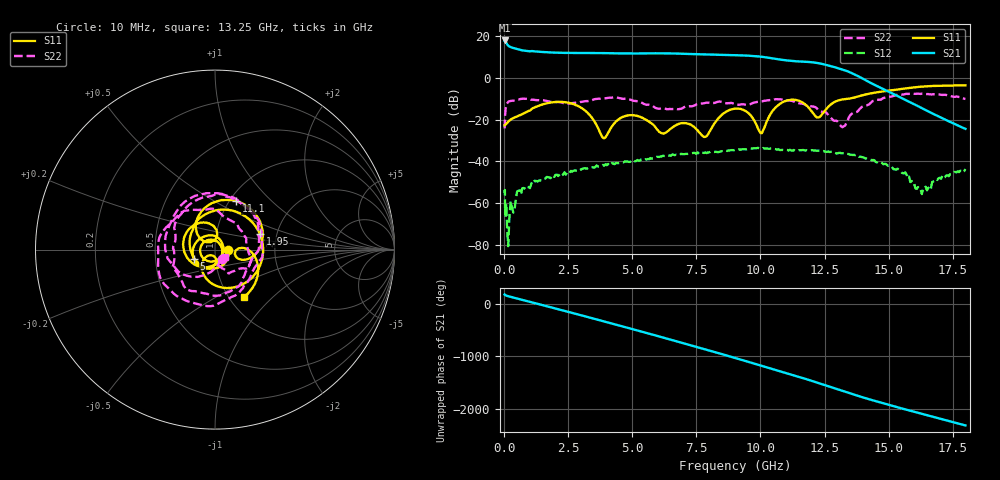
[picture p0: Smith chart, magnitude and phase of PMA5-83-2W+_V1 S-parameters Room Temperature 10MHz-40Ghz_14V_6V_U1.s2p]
!Mini-Circuits Laboratory
!S-Parameters
!Model: US-AMP-1
!Run / Lot / Date Code: N/A /  / N/A
!Fixture: ON TB-
!Network Analyzer: NFA N8975A;  Serial number: 74408
!Date: 12/1/2023 at 8:03:47 AM
!No.: Unit# 1 (#1)
!Tested with:
!Condition 4: Vdd = +14V; Vg2= +6V; Idd= 400mA
# Hz  S  dB  R  50
!Frequency  S11 dB  S11 Deg  S21 dB  S21 Deg  S12 dB  S12 Deg  S22 dB  S22 Deg
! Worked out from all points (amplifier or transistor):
!   368 points, 10 MHz to 18 GHz, reference 50 ohm
!   highest |S21| = 18.0 dB at 20 MHz (marker M1)
!   |S21| within 3 dB of that: start of sweep to 215.1 MHz
!   unconditionally stable (mu >= 1): start of sweep to end of sweep
!   at 2.7 GHz: K = 18.48, MAG = 12.5 dB, |S12| = -44.4 dB
!   at 8.85 GHz: K = 6.93, MAG = 11.4 dB, |S12| = -34.6 dB
!   at 18 GHz: K = 621.43, MAG = -21.3 dB, |S12| = -43.6 dB
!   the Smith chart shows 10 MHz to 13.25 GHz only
!   S11 on the Smith chart (normalised r, x): 10 MHz: 1.16, -0.00; 1.95 GHz: 1.64, +0.30; 5 GHz: 0.78, -0.08; 11.1 GHz: 1.07, +0.64; 13.25 GHz: 1.18, -0.68
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1e7  -22.71 -0.8  17.78 177.5  -55.13 12.2  -24.12 -54.2
2e7  -22.66 -4.0  17.98 174.2  -53.64 12.2  -20.38 -83.6
5e8  -18.43 -141.9  13.87 101.3  -54.33 60.9  -10.56 141.3
1.1e9  -14.54 124.1  12.89 26.5  -49.30 -38.3  -10.36 74.3
1.95e9  -11.53 18.7  12.15 -82.2  -47.38 -143.6  -11.66 1.0
2.55e9  -11.99 -46.9  12.01 -158.9  -45.44 143.8  -12.18 -34.4
3.05e9  -14.67 -98.4  12.00 136.4  -43.49 80.3  -11.31 -59.1
4.05e9  -26.31 -85.6  11.88 4.8  -41.17 -44.7  -9.50 -129.6
5e9  -17.81 -157.0  11.73 -120.2  -40.01 -165.1  -10.77 150.6
5.5e9  -19.78 142.5  11.79 173.5  -38.90 132.6  -12.63 106.6
6.05e9  -25.82 33.7  11.82 99.3  -37.81 62.9  -14.69 60.9
6.75e9  -22.28 -127.2  11.68 3.4  -36.87 -27.7  -14.91 15.3
7.4e9  -23.37 130.0  11.42 -85.6  -35.87 -112.1  -13.24 -41.0
8.15e9  -22.79 -78.0  11.17 171.3  -35.36 151.0  -11.98 -105.3
9.05e9  -14.66 152.7  10.89 45.0  -34.50 28.8  -12.78 -168.8
9.95e9  -25.36 91.9  10.30 -86.1  -33.76 -96.6  -11.33 140.5
1.05e10  -15.35 129.0  9.34 -166.6  -33.84 -172.3  -10.48 94.0
1.11e10  -10.61 66.3  8.32 108.1  -34.72 104.3  -10.70 42.8
1.205e10  -16.92 -21.3  7.47 -33.1  -34.63 -31.5  -13.64 -29.3
1.325e10  -10.20 -57.9  3.87 136.8  -36.07 138.5  -23.11 -38.9
1.505e10  -6.00 124.2  -6.83 -127.1  -41.97 -105.9  -8.95 -117.5
1.8e10  -3.50 177.6  -24.35 -154.2  -43.58 83.8  -10.04 57.3
